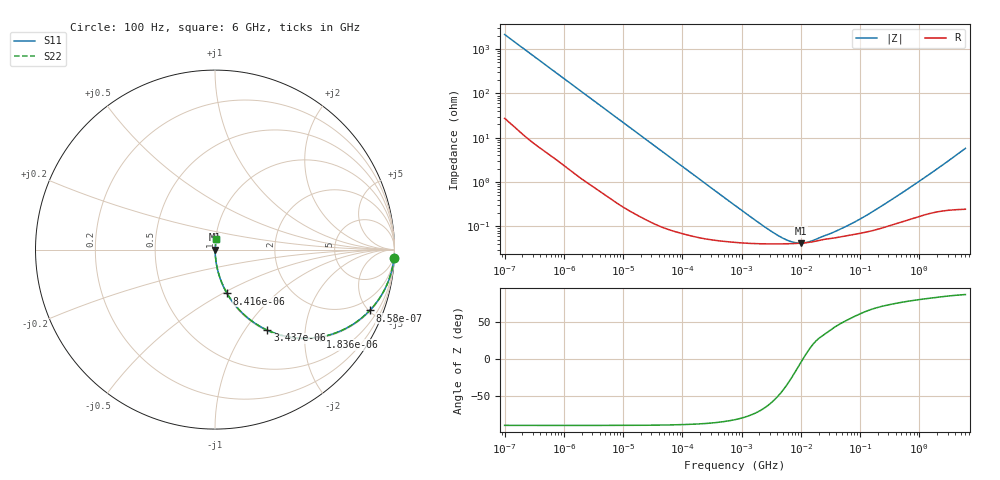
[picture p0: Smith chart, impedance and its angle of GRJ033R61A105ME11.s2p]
!Murata Part Number: GRJ033R61A105ME11
!These Parameters are Measured in Series Mode Connection
!Data Generated on Jun 19, 2026
!  o--ll--o
!Port1  Port2
!  o------o
!Operation Temp=25[degC], DC Bias Voltage=0[V]
!Freq. Start=100[Hz] Stop=6[GHz] 401[Steps]
# Hz S RI R 50
!Freq.(Hz) S11(Real) S11(Imag) S21(Real) S21(Imag) S12(Real) S12(Imag) S22(Real) S22(Imag)
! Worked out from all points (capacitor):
!   401 points, 100 Hz to 6 GHz, reference 50 ohm
!   read as one part in series: C = 740 nF near 109 Hz
!   lowest |Z| = 42.1 mohm at 9.942 MHz (marker M1)
!   series resonance near 10.77 MHz, so ESL is about 290 pH
!   S11 on the Smith chart (normalised r, x): 100 Hz: 2, -43; 858 Hz: 1.06, -5.07; 1.836 kHz: 1.03, -2.38; 3.437 kHz: 1.01, -1.28; 8.416 kHz: 1.01, -0.52; 6 GHz: 1.00, +0.12
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100  0.9972 -0.0465  0.00277 0.0465  0.00277 0.0465  0.9972 -0.0465
320  0.977 -0.1446  0.023 0.1446  0.023 0.1446  0.977 -0.1446
548  0.9377 -0.2364  0.0623 0.2364  0.0623 0.2364  0.9377 -0.2364
858  0.8627 -0.3387  0.1373 0.3387  0.1373 0.3387  0.8627 -0.3387
1227  0.7571 -0.4235  0.2429 0.4235  0.2429 0.4235  0.7571 -0.4235
1836  0.5855 -0.4873  0.4145 0.4873  0.4145 0.4873  0.5855 -0.4873
2008  0.5422 -0.4929  0.4578 0.4929  0.4578 0.4929  0.5422 -0.4929
3437  0.2919 -0.449  0.7081 0.449  0.7081 0.449  0.2919 -0.449
5378  0.1465 -0.3478  0.8535 0.3478  0.8535 0.3478  0.1465 -0.3478
8416  0.067 -0.2441  0.933 0.2441  0.933 0.2441  0.067 -0.2441
17227  0.018 -0.1262  0.982 0.1262  0.982 0.1262  0.018 -0.1262
40335  0.00407 -0.055  0.9959 0.055  0.9959 0.055  0.00407 -0.055
123542  0.00097 -0.0182  0.999 0.0182  0.999 0.0182  0.00097 -0.0182
774597  0.000445 -0.00294  0.9996 0.00294  0.9996 0.00294  0.000445 -0.00294
4246196  0.000404 -0.000458  0.9996 0.000458  0.9996 0.000458  0.000404 -0.000458
6644369  0.000408 -0.000214  0.9996 0.000214  0.9996 0.000214  0.000408 -0.000214
9941735  0.000419 -3.37e-05  0.9996 3.37e-05  0.9996 3.37e-05  0.000419 -3.37e-05
1.555665e7  0.000449 0.000154  0.9996 -0.000154  0.9996 -0.000154  0.000449 0.000154
3.482834e7  0.000543 0.000487  0.9995 -0.000487  0.9995 -0.000487  0.000543 0.000487
7.455971e7  0.000653 0.000991  0.9993 -0.000991  0.9993 -0.000991  0.000653 0.000991
3.124326e8  0.00105 0.00359  0.999 -0.00359  0.999 -0.00359  0.00105 0.00359
6e9  0.00573 0.0572  0.9943 -0.0572  0.9943 -0.0572  0.00573 0.0572
